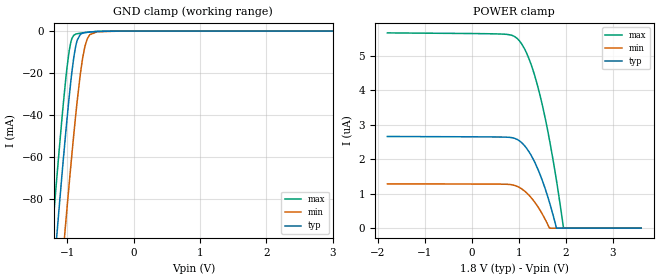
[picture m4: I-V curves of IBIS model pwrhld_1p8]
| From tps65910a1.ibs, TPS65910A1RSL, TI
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|   pwrhld_1p8 Model
[Model]   pwrhld_1p8
Model_type   Input
Vinl = 0.45
Vinh = 1.3
|   typ   min   max
|   (nom PVT)   (fast PVT)   (slow PVT)
C_comp   1.767e-13   1.755e-13   1.788e-13
| Where nom  PVT is Nominal Process, 1.8V, 27C
|   Fast PVT is Strong Process,  1.95V, -40C
|   Slow PVT is Weak Process,   1.65V, 125C
[Voltage Range]   1.8   1.65   1.95
|Junction Temperature
[Temperature Range]   27   125   -40
[Power Clamp Reference]   1.8   1.65   1.95
[GND Clamp Reference]   0   0   0
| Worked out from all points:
|   GND clamp passes 1 mA (typ) near -0.77 V on its own axis
[GND Clamp]
|   Voltage   I(typ)   I(min)   I(max)
-1.8V     -355.8mA   -398.5mA   -329.8mA
-1.249V   -133.5mA   -177.7mA   -106mA
-1.203V   -115.8mA   -160mA     -88.24mA
-1.166V   -101.6mA   -145.8mA   -74.13mA
-1.121V   -84.63mA   -128.6mA   -57.33mA
-1.016V   -46.8mA    -89.59mA   -21.56mA
-945mV    -24.17mA   -64.38mA   -5.393mA
-873mV    -7.569mA   -40.75mA   -1.478mA
-801.6mV  -1.617mA   -20.69mA   -993.5uA
-731.4mV  -727.5uA   -7.216mA   -698.1uA
-546mV    -167.1uA   -305.9uA   -128uA
3.6V      0A         0A         0A
[POWER Clamp]
|   Voltage   I(typ)   I(min)   I(max)
-1.8V     2.663uA    1.287uA    5.672uA
594.6mV   2.647uA    1.278uA    5.64uA
830.1mV   2.633uA    1.264uA    5.61uA
963.7mV   2.577uA    1.213uA    5.509uA
1.115V    2.404uA    1.084uA    5.221uA
1.217V    2.215uA    954nA      4.913uA
1.337V    1.914uA    753.4nA    4.426uA
1.458V    1.529uA    502.2nA    3.808uA
1.652V    743.3nA    0A         2.556uA
1.798V    0A         0A         1.395uA
1.95V     0A         0A         0A
3.6V      0A         0A         0A
